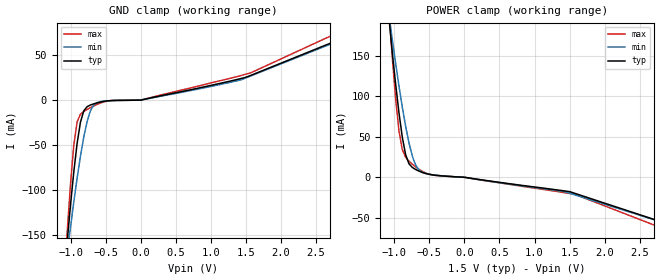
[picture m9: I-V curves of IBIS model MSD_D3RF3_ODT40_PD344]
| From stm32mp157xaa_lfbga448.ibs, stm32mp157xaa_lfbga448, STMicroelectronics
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[Model] MSD_D3RF3_ODT40_PD344
Model_type   Input
C_comp 2.224pF   2.184pF   2.300pF
Vinh = 925.000mV
Vinl = 575.000mV
[Temperature Range]   25.000   125.000   -40.000
[Voltage Range]   1.500V   1.425V   1.575V
[GND Clamp Reference]   0.00V   0.00V   0.00V
[POWER Clamp Reference]   1.500V   1.425V   1.575V
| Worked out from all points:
|   GND clamp passes 1 mA (typ) near -0.49 V on its own axis
|   POWER clamp passes 1 mA (typ) near -0.21 V on its own axis
[GND Clamp]
-1.48V    -588.7mA   -456.5mA   -787.5mA
-1.05V    -158.8mA   -171.3mA   -148.9mA
-1.002V   -117.5mA   -141.8mA   -94.47mA
-954.6mV  -80.12mA   -113.5mA   -50.47mA
-906.8mV  -48.24mA   -86.77mA   -24.24mA
-859.1mV  -24.58mA   -62.37mA   -15.62mA
-763.6mV  -7.292mA   -23.61mA   -10.37mA
-715.9mV  -5.39mA    -11.68mA   -8.33mA
-620.5mV  -3.036mA   -2.788mA   -4.71mA
900nV     15.63nA    14.14nA    18.4nA
1.575V    27.59mA    26.98mA    30.44mA
2.959V    71.09mA    69.9mA     80.09mA
[Power Clamp]
-1.459V   582.1mA    457.9mA    771.2mA
-1.077V   197.1mA    200.9mA    207.3mA
-1.03V    154.7mA    170.5mA    149.3mA
-981.8mV  115.5mA    141mA      97.62mA
-934.1mV  79.91mA    112.9mA    57.39mA
-886.4mV  49.61mA    86.67mA    34.22mA
-838.6mV  27.8mA     62.95mA    24.69mA
-743.2mV  12.11mA    26.03mA    16.05mA
-647.7mV  7.55mA     8.901mA    9.729mA
-552.3mV  4.621mA    4.628mA    5.276mA
1.548V    -19.08mA   -20.97mA   -20.65mA
2.98V     -59.82mA   -59.79mA   -68.11mA
